| Texas Instruments Incorporated
| ADS8555: 16-Bit, Six-Channel, Simultaneous Sampling ADC
| ADS8556: 16-Bit, Six-Channel, Simultaneous Sampling ADC
| ADS8557: 14-Bit, Six-Channel, Simultaneous Sampling ADC
| ADS8558: 12-Bit, Six-Channel, Simultaneous Sampling ADC
| Marketing part#   Voltage Range   Package-type   #pins/pkg drawing
| ADS855XPM   2.7V - 5.5V   SQFP   64-pin PM
| Package Dimension   Width   Length   Height
|   346.0mm   346.0mm   41.0mm
[IBIS ver]   4.1
[File name]   ads855x.ibs
[File Rev]   1.0
[Date]   11/16/2010
[Source]   Texas Instruments Incorporated.
   Analog-eLab, HPA
   12500 TI Blvd
   Dallas, TX -75243
   e-mail: elab_ibis@list.ti.com
[Notes]   Revision History
   Rev 1.0: 09/16/2009
   - Initial version of the model
   - Model based on simulations from TIspiceD
   - Model not matched to measurements
   - min C_comp was obtained at corner high BVDD, low  temperature, strong process
   - max C_comp was obtained at corner low  BVDD, high temperature, weak process
   Rev 2.0: 11/16/2010
   Components ADS8557 and ADS8558 were added
   Rev 3.0: 11/30/2010
   - Added ADS8555 product family to this IBIS model file
[Disclaimer] This product is designed as an aid for customers of Texas
   Instruments.
   No warranties, either expressed or implied, with respect
   to this third party software (if any) or with respect to
   its fitness for any particular purpose is claimed by Texas
   Instruments or the author. The software (if any) is provided
   solely on an "as is" basis. The entire risk as to its quality
   and performance is with the customer.
[Copyright]   (C)Copyright 2010 Texas Instruments Incorporated.
   All rights reserved.
|  Component ADS8555, ADS8556: 16-Bit, Six-Channel, Simultaneous Sampling ADC
[Component]   ADS8555_6
[Manufacturer]  Texas Instruments Incorporated
[Package]   |64-pin SQFP PM package
|   typ   min   max
R_pkg   0.013   0.013   0.014
L_pkg   1.951nH   1.787nH   2.164nH
C_pkg   0.403pF   0.347pF   0.445pF
[Pin] signal_name   model_name   R_pin   L_pin   C_pin
|   Ohm   Henry   Farad
   1  DB14/REFBUFEN DIO   0.01375  2.16404E-09  0.36893E-12
   2  DB13/SDIN   DIO   0.01364  2.06651E-09  0.44422E-12
   3  DB12   DIO   0.01327  1.98992E-09  0.43874E-12
   4  DB11   DIO   0.01305  1.94514E-09  0.41947E-12
   5  DB10/SDO_C   DIO   0.01314  1.91793E-09  0.41193E-12
   6  DB9/SDO_B   DIO   0.01277  1.85279E-09  0.39172E-12
   7  DB8/SDO_A   DIO   0.01239  1.79219E-09  0.38069E-12
   8  BGND   GND   0.01228  1.78659E-09  0.34665E-12
   9  BVDD   POWER   0.01229  1.78696E-09  0.34655E-12
   10  DB7/HBEN/DCEN DIO   0.01238  1.79227E-09  0.38064E-12
   11  DB6/SCLK   DIO   0.01278  1.85346E-09  0.39156E-12
   12  DB5/DCIN_A   DIO   0.01314  1.91809E-09  0.41197E-12
   13  DB4/DCIN_B   DIO   0.01305  1.94507E-09  0.41976E-12
   14  DB3/DCIN_C   DIO   0.01326  1.98949E-09  0.43931E-12
   15  DB2/SEL_C   DIO   0.01363  2.06569E-09  0.44472E-12
   16  DB1/SEL_B   DIO   0.01375  2.16395E-09  0.36892E-12
   17  DB0/SEL_A   DIO   0.01375  2.16405E-09  0.36893E-12
   18  BUSY/INT   DOUT   0.01364  2.06651E-09  0.44422E-12
   19  CS/FS   DIN   0.01327  1.98992E-09  0.43874E-12
   20  RD_BAR   DIN   0.01305  1.94514E-09  0.41948E-12
   21  CONVST_C   DIN   0.01314  1.91793E-09  0.41193E-12
   22  CONVST_B   DIN   0.01277  1.85279E-09  0.39171E-12
   23  CONVST_A   DIN   0.01239  1.79219E-09  0.38069E-12
   24  STBY_BAR   DIN   0.01228  1.78659E-09  0.34665E-12
   25  AGND   GND   0.01229  1.78695E-09  0.34656E-12
   26  AVDD   POWER   0.01238  1.79225E-09  0.38065E-12
   27  RANGE/XCLK   DIO   0.01278  1.85345E-09  0.39156E-12
   28  RESET   DIN   0.01314  1.91809E-09  0.41197E-12
   29  WORD/BYTE   DIN   0.01305  1.94504E-09  0.41979E-12
   30  HVSS   GND   0.01326  1.98925E-09  0.43938E-12   |negative power supply
   31  HVDD   POWER   0.01363  2.06564E-09  0.44475E-12
   32  NC   NC   0.01374  2.16370E-09  0.36899E-12
   33  CH_A0   TERM   0.01375  2.16404E-09  0.36893E-12   |AI
   34  NC   NC   0.01364  2.06651E-09  0.44422E-12
   35  NC   NC   0.01327  1.98992E-09  0.43874E-12
   36  CH_A1   TERM   0.01305  1.94514E-09  0.41947E-12   |AI
   37  NC   NC   0.01314  1.91793E-09  0.41193E-12
   38  NC   NC   0.01277  1.85279E-09  0.39172E-12
   39  CH_B0   TERM   0.01239  1.79219E-09  0.38069E-12   |AI
   40  NC   NC   0.01228  1.78659E-09  0.34665E-12
   41  NC   NC   0.01229  1.78696E-09  0.34655E-12
   42  CH_B1   TERM   0.01238  1.79227E-09  0.38064E-12   |AI
   43  NC   NC   0.01278  1.85346E-09  0.39156E-12
   44  NC   NC   0.01314  1.91809E-09  0.41197E-12
   45  CH_C0   TERM   0.01305  1.94507E-09  0.41976E-12   |AI
   46  NC   NC   0.01326  1.98949E-09  0.43931E-12
   47  NC   NC   0.01363  2.06569E-09  0.44472E-12
   48  CH_C1   TERM   0.01375  2.16395E-09  0.36892E-12   |AI
   49  NC   NC   0.01375  2.16406E-09  0.36893E-12
   50  NC   NC   0.01364  2.06651E-09  0.44422E-12
   51  REFIO   TERM   0.01327  1.98992E-09  0.43874E-12   |AIO
   52  NC   NC   0.01305  1.94512E-09  0.41948E-12
   53  NC   NC   0.01314  1.91793E-09  0.41193E-12
   54  REFC_A   TERM   0.01277  1.85279E-09  0.39171E-12   |AI
   55  NC   NC   0.01239  1.79219E-09  0.38069E-12
   56  REFC_B   TERM   0.01228  1.78659E-09  0.34665E-12   |AI
   57  NC   NC   0.01229  1.78695E-09  0.34656E-12
   58  REFC_C   TERM   0.01238  1.79225E-09  0.38065E-12   |AI
   59  NC   NC   0.01278  1.85345E-09  0.39156E-12
   60  NC   NC   0.01314  1.91809E-09  0.41197E-12
   61  PAR/SER   DIN   0.01305  1.94504E-09  0.41979E-12
   62  HW/SW   DIN   0.01326  1.98925E-09  0.43938E-12
   63  REFEN/WR   DIN   0.01363  2.06564E-09  0.44475E-12
   64  DB15   DIO   0.01374  2.16370E-09  0.36899E-12
|  Component ADS8557: 14-Bit, Six-Channel, Simultaneous Sampling ADC
[Component]   ADS8557
[Manufacturer]  Texas Instruments Incorporated
[Package]   |64-pin SQFP PM package
|   typ   min   max
R_pkg   0.013   0.013   0.014
L_pkg   1.951nH   1.787nH   2.164nH
C_pkg   0.403pF   0.347pF   0.445pF
[Pin] signal_name   model_name   R_pin   L_pin   C_pin
|   Ohm   Henry   Farad
   1  DB14/REFBUFEN DIO   0.01375  2.16404E-09  0.36893E-12
   2  DB13/SDIN   DIO   0.01364  2.06651E-09  0.44422E-12
   3  DB12   DIO   0.01327  1.98992E-09  0.43874E-12
   4  DB11   DIO   0.01305  1.94514E-09  0.41947E-12
   5  DB10/SDO_C   DIO   0.01314  1.91793E-09  0.41193E-12
   6  DB9/SDO_B   DIO   0.01277  1.85279E-09  0.39172E-12
   7  DB8/SDO_A   DIO   0.01239  1.79219E-09  0.38069E-12
   8  BGND   GND   0.01228  1.78659E-09  0.34665E-12
   9  BVDD   POWER   0.01229  1.78696E-09  0.34655E-12
   10  DB7/HBEN/DCEN DIO   0.01238  1.79227E-09  0.38064E-12
   11  DB6/SCLK   DIO   0.01278  1.85346E-09  0.39156E-12
   12  DB5/DCIN_A   DIO   0.01314  1.91809E-09  0.41197E-12
   13  DB4/DCIN_B   DIO   0.01305  1.94507E-09  0.41976E-12
   14  DB3/DCIN_C   DIO   0.01326  1.98949E-09  0.43931E-12
   15  DB2/SEL_C   DIO   0.01363  2.06569E-09  0.44472E-12
   16  DB1/SEL_B   DIO   0.01375  2.16395E-09  0.36892E-12
   17  DB0/SEL_A   DIO   0.01375  2.16405E-09  0.36893E-12
   18  BUSY/INT   DOUT   0.01364  2.06651E-09  0.44422E-12
   19  CS/FS   DIN   0.01327  1.98992E-09  0.43874E-12
   20  RD_BAR   DIN   0.01305  1.94514E-09  0.41948E-12
   21  CONVST_C   DIN   0.01314  1.91793E-09  0.41193E-12
   22  CONVST_B   DIN   0.01277  1.85279E-09  0.39171E-12
   23  CONVST_A   DIN   0.01239  1.79219E-09  0.38069E-12
   24  STBY_BAR   DIN   0.01228  1.78659E-09  0.34665E-12
   25  AGND   GND   0.01229  1.78695E-09  0.34656E-12
   26  AVDD   POWER   0.01238  1.79225E-09  0.38065E-12
   27  RANGE/XCLK   DIO   0.01278  1.85345E-09  0.39156E-12
   28  RESET   DIN   0.01314  1.91809E-09  0.41197E-12
   29  WORD/BYTE   DIN   0.01305  1.94504E-09  0.41979E-12
   30  HVSS   GND   0.01326  1.98925E-09  0.43938E-12   |negative power supply
   31  HVDD   POWER   0.01363  2.06564E-09  0.44475E-12
   32  NC   NC   0.01374  2.16370E-09  0.36899E-12
   33  CH_A0   TERM   0.01375  2.16404E-09  0.36893E-12   |AI
   34  NC   NC   0.01364  2.06651E-09  0.44422E-12
   35  NC   NC   0.01327  1.98992E-09  0.43874E-12
   36  CH_A1   TERM   0.01305  1.94514E-09  0.41947E-12   |AI
   37  NC   NC   0.01314  1.91793E-09  0.41193E-12
   38  NC   NC   0.01277  1.85279E-09  0.39172E-12
   39  CH_B0   TERM   0.01239  1.79219E-09  0.38069E-12   |AI
   40  NC   NC   0.01228  1.78659E-09  0.34665E-12
   41  NC   NC   0.01229  1.78696E-09  0.34655E-12
   42  CH_B1   TERM   0.01238  1.79227E-09  0.38064E-12   |AI
   43  NC   NC   0.01278  1.85346E-09  0.39156E-12
   44  NC   NC   0.01314  1.91809E-09  0.41197E-12
   45  CH_C0   TERM   0.01305  1.94507E-09  0.41976E-12   |AI
   46  NC   NC   0.01326  1.98949E-09  0.43931E-12
   47  NC   NC   0.01363  2.06569E-09  0.44472E-12
   48  CH_C1   TERM   0.01375  2.16395E-09  0.36892E-12   |AI
   49  NC   NC   0.01375  2.16406E-09  0.36893E-12
   50  NC   NC   0.01364  2.06651E-09  0.44422E-12
   51  REFIO   TERM   0.01327  1.98992E-09  0.43874E-12   |AIO
   52  NC   NC   0.01305  1.94512E-09  0.41948E-12
   53  NC   NC   0.01314  1.91793E-09  0.41193E-12
   54  REFC_A   TERM   0.01277  1.85279E-09  0.39171E-12   |AI
   55  NC   NC   0.01239  1.79219E-09  0.38069E-12
   56  REFC_B   TERM   0.01228  1.78659E-09  0.34665E-12   |AI
   57  NC   NC   0.01229  1.78695E-09  0.34656E-12
   58  REFC_C   TERM   0.01238  1.79225E-09  0.38065E-12   |AI
   59  NC   NC   0.01278  1.85345E-09  0.39156E-12
   60  NC   NC   0.01314  1.91809E-09  0.41197E-12
   61  PAR/SER   DIN   0.01305  1.94504E-09  0.41979E-12
   62  HW/SW   DIN   0.01326  1.98925E-09  0.43938E-12
   63  REFEN/WR   DIN   0.01363  2.06564E-09  0.44475E-12
   64  DB15   DIO   0.01374  2.16370E-09  0.36899E-12
|  Component ADS8558: 12-Bit, Six-Channel, Simultaneous Sampling ADC
[Component]   ADS8558
[Manufacturer]  Texas Instruments Incorporated
[Package]   |64-pin SQFP PM package
|   typ   min   max
R_pkg   0.013   0.013   0.014
L_pkg   1.951nH   1.787nH   2.164nH
C_pkg   0.403pF   0.347pF   0.445pF
[Pin] signal_name   model_name   R_pin   L_pin   C_pin
|   Ohm   Henry   Farad
   1  DB14/REFBUFEN DIO   0.01375  2.16404E-09  0.36893E-12
   2  DB13/SDIN   DIO   0.01364  2.06651E-09  0.44422E-12
   3  DB12   DIO   0.01327  1.98992E-09  0.43874E-12
   4  DB11   DIO   0.01305  1.94514E-09  0.41947E-12
   5  DB10/SDO_C   DIO   0.01314  1.91793E-09  0.41193E-12
   6  DB9/SDO_B   DIO   0.01277  1.85279E-09  0.39172E-12
   7  DB8/SDO_A   DIO   0.01239  1.79219E-09  0.38069E-12
   8  BGND   GND   0.01228  1.78659E-09  0.34665E-12
   9  BVDD   POWER   0.01229  1.78696E-09  0.34655E-12
   10  DB7/HBEN/DCEN DIO   0.01238  1.79227E-09  0.38064E-12
   11  DB6/SCLK   DIO   0.01278  1.85346E-09  0.39156E-12
   12  DB5/DCIN_A   DIO   0.01314  1.91809E-09  0.41197E-12
   13  DB4/DCIN_B   DIO   0.01305  1.94507E-09  0.41976E-12
   14  DB3/DCIN_C   DIO   0.01326  1.98949E-09  0.43931E-12
   15  DB2/SEL_C   DIO   0.01363  2.06569E-09  0.44472E-12
   16  DB1/SEL_B   DIO   0.01375  2.16395E-09  0.36892E-12
   17  DB0/SEL_A   DIO   0.01375  2.16405E-09  0.36893E-12
   18  BUSY/INT   DOUT   0.01364  2.06651E-09  0.44422E-12
   19  CS/FS   DIN   0.01327  1.98992E-09  0.43874E-12
   20  RD_BAR   DIN   0.01305  1.94514E-09  0.41948E-12
   21  CONVST_C   DIN   0.01314  1.91793E-09  0.41193E-12
   22  CONVST_B   DIN   0.01277  1.85279E-09  0.39171E-12
   23  CONVST_A   DIN   0.01239  1.79219E-09  0.38069E-12
   24  STBY_BAR   DIN   0.01228  1.78659E-09  0.34665E-12
   25  AGND   GND   0.01229  1.78695E-09  0.34656E-12
   26  AVDD   POWER   0.01238  1.79225E-09  0.38065E-12
   27  RANGE/XCLK   DIO   0.01278  1.85345E-09  0.39156E-12
   28  RESET   DIN   0.01314  1.91809E-09  0.41197E-12
   29  WORD/BYTE   DIN   0.01305  1.94504E-09  0.41979E-12
   30  HVSS   GND   0.01326  1.98925E-09  0.43938E-12   |negative power supply
   31  HVDD   POWER   0.01363  2.06564E-09  0.44475E-12
   32  NC   NC   0.01374  2.16370E-09  0.36899E-12
   33  CH_A0   TERM   0.01375  2.16404E-09  0.36893E-12   |AI
   34  NC   NC   0.01364  2.06651E-09  0.44422E-12
   35  NC   NC   0.01327  1.98992E-09  0.43874E-12
   36  CH_A1   TERM   0.01305  1.94514E-09  0.41947E-12   |AI
   37  NC   NC   0.01314  1.91793E-09  0.41193E-12
   38  NC   NC   0.01277  1.85279E-09  0.39172E-12
   39  CH_B0   TERM   0.01239  1.79219E-09  0.38069E-12   |AI
   40  NC   NC   0.01228  1.78659E-09  0.34665E-12
   41  NC   NC   0.01229  1.78696E-09  0.34655E-12
   42  CH_B1   TERM   0.01238  1.79227E-09  0.38064E-12   |AI
   43  NC   NC   0.01278  1.85346E-09  0.39156E-12
   44  NC   NC   0.01314  1.91809E-09  0.41197E-12
   45  CH_C0   TERM   0.01305  1.94507E-09  0.41976E-12   |AI
   46  NC   NC   0.01326  1.98949E-09  0.43931E-12
   47  NC   NC   0.01363  2.06569E-09  0.44472E-12
   48  CH_C1   TERM   0.01375  2.16395E-09  0.36892E-12   |AI
   49  NC   NC   0.01375  2.16406E-09  0.36893E-12
   50  NC   NC   0.01364  2.06651E-09  0.44422E-12
   51  REFIO   TERM   0.01327  1.98992E-09  0.43874E-12   |AIO
   52  NC   NC   0.01305  1.94512E-09  0.41948E-12
   53  NC   NC   0.01314  1.91793E-09  0.41193E-12
   54  REFC_A   TERM   0.01277  1.85279E-09  0.39171E-12   |AI
   55  NC   NC   0.01239  1.79219E-09  0.38069E-12
   56  REFC_B   TERM   0.01228  1.78659E-09  0.34665E-12   |AI
   57  NC   NC   0.01229  1.78695E-09  0.34656E-12
   58  REFC_C   TERM   0.01238  1.79225E-09  0.38065E-12   |AI
   59  NC   NC   0.01278  1.85345E-09  0.39156E-12
   60  NC   NC   0.01314  1.91809E-09  0.41197E-12
   61  PAR/SER   DIN   0.01305  1.94504E-09  0.41979E-12
   62  HW/SW   DIN   0.01326  1.98925E-09  0.43938E-12
   63  REFEN/WR   DIN   0.01363  2.06564E-09  0.44475E-12
   64  DB15   DIO   0.01374  2.16370E-09  0.36899E-12
[Pin Mapping]pulldown_ref pullup_ref gnd_clamp_ref power_clamp_ref
|   GNDBUS1 is BGND,   PWRBUS1 is  BVDD
 1   GNDBUS1   PWRBUS1   GNDBUS1   PWRBUS1  | DIO
 2   GNDBUS1   PWRBUS1   GNDBUS1   PWRBUS1  | DIO
 3   GNDBUS1   PWRBUS1   GNDBUS1   PWRBUS1  | DIO
 4   GNDBUS1   PWRBUS1   GNDBUS1   PWRBUS1  | DIO
 5   GNDBUS1   PWRBUS1   GNDBUS1   PWRBUS1  | DIO
 6   GNDBUS1   PWRBUS1   GNDBUS1   PWRBUS1  | DIO
 7   GNDBUS1   PWRBUS1   GNDBUS1   PWRBUS1  | DIO
 8   GNDBUS1   NC   | BGND
 9   NC   PWRBUS1   | BVDD
10   GNDBUS1   PWRBUS1   GNDBUS1   PWRBUS1  | DIO
11   GNDBUS1   PWRBUS1   GNDBUS1   PWRBUS1  | DIO
12   GNDBUS1   PWRBUS1   GNDBUS1   PWRBUS1  | DIO
13   GNDBUS1   PWRBUS1   GNDBUS1   PWRBUS1  | DIO
14   GNDBUS1   PWRBUS1   GNDBUS1   PWRBUS1  | DIO
15   GNDBUS1   PWRBUS1   GNDBUS1   PWRBUS1  | DIO
16   GNDBUS1   PWRBUS1   GNDBUS1   PWRBUS1  | DIO
17   GNDBUS1   PWRBUS1   GNDBUS1   PWRBUS1  | DIO
18   GNDBUS1   PWRBUS1   NC   NC   | DOUT
19   NC   NC   GNDBUS1   PWRBUS1  | DIN
20   NC   NC   GNDBUS1   PWRBUS1  | DIN
21   NC   NC   GNDBUS1   PWRBUS1  | DIN
22   NC   NC   GNDBUS1   PWRBUS1  | DIN
23   NC   NC   GNDBUS1   PWRBUS1  | DIN
24   NC   NC   GNDBUS1   PWRBUS1  | DIN
25   GNDBUS2   NC   | AGND
26   NC   PWRBUS2   | AVDD
27   GNDBUS1   PWRBUS1   GNDBUS1   PWRBUS1  | DIO
28   NC   NC   GNDBUS1   PWRBUS1  | DIN
29   NC   NC   GNDBUS1   PWRBUS1  | DIN
30   GNDBUS3   NC   | HVSS, negative power supply
31   NC   PWRBUS3   | HVDD
32   NC   NC   NC   NC   | NC
33   NC   NC   NC   NC   | AI
34   NC   NC   NC   NC   | NC
35   NC   NC   NC   NC   | NC
36   NC   NC   NC   NC   | AI
37   NC   NC   NC   NC   | NC
38   NC   NC   NC   NC   | NC
39   NC   NC   NC   NC   | AI
40   NC   NC   NC   NC   | NC
41   NC   NC   NC   NC   | NC
42   NC   NC   NC   NC   | AI
43   NC   NC   NC   NC   | NC
44   NC   NC   NC   NC   | NC
45   NC   NC   NC   NC   | AI
46   NC   NC   NC   NC   | NC
47   NC   NC   NC   NC   | NC
48   NC   NC   NC   NC   | AI
49   NC   NC   NC   NC   | NC
50   NC   NC   NC   NC   | NC
51   NC   NC   NC   NC   | AIO
52   NC   NC   NC   NC   | NC
53   NC   NC   NC   NC   | NC
54   NC   NC   NC   NC   | AI
55   NC   NC   NC   NC   | NC
56   NC   NC   NC   NC   | AI
57   NC   NC   NC   NC   | NC
58   NC   NC   NC   NC   | AI
59   NC   NC   NC   NC   | NC
60   NC   NC   NC   NC   | NC
61   NC   NC   GNDBUS1   PWRBUS1  | DIN
62   NC   NC   GNDBUS1   PWRBUS1  | DIN
63   NC   NC   GNDBUS1   PWRBUS1  | DIN
64   GNDBUS1   PWRBUS1   GNDBUS1   PWRBUS1  | DIO
[Model Selector]   DIN
DIN_3   2.70V - 3.30V Input Model
DIN_5   4.50V - 5.50V Input Model
[Model Selector]   DIO
DIO_3   2.70V - 3.30V DIO Model
DIO_5   4.50V - 5.50V DIO Model
[Model Selector]   DOUT
DOUT_3   2.70V - 3.30V Output Model
DOUT_5   4.50V - 5.50V Output Model
[Model] TERM
Model_type Terminator
C_comp   0  0  0
| variable   typ   min   max
[Voltage Range]   15.0000V  5.0000V   16.5000V  |min value= 2 * VREF
[POWER Clamp Reference]  15.0000V  5.0000V   16.5000V  |min value= 2 * VREF
[GND Clamp Reference]   0.00000V  0.0000V   0.0000V
[Temperature Range]   40   125   -40
| Models and submodels in the file (7): TERM (Terminator), DIN_3 (Input), DIN_5 (Input), DIO_3 (I/O), DIO_5 (I/O), DOUT_3 (Output), DOUT_5 (Output)
